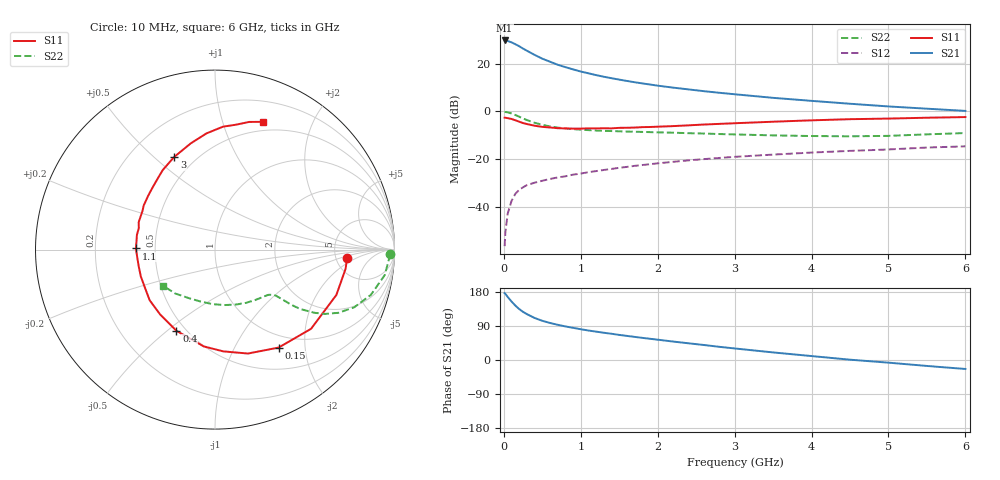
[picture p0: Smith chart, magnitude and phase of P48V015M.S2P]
! SIEMENS Small Signal Semiconductors
! BFP182
! Si NPN RF Bipolar Junction Transistor in SOT143
! VCE = 8 V  IC = 15 mA
! Common Emitter S-Parameters:  March  1996
# GHz  S  MA  R  50
!  f  S11  S21  S12  S22
! GHz  MAG  ANG  MAG  ANG  MAG  ANG  MAG  ANG
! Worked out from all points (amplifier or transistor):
!   36 points, 10 MHz to 6 GHz, reference 50 ohm
!   highest |S21| = 29.7 dB at 10 MHz (marker M1)
!   |S21| within 3 dB of that: start of sweep to 229 MHz
!   unconditionally stable (mu >= 1): 1.087 GHz to 5.576 GHz
!   at 250 MHz: K = 0.39, MSG = 29.1 dB, |S12| = -31.8 dB
!   at 1.4 GHz: K = 1.09, MAG = 17.1 dB, |S12| = -24.1 dB
!   at 6 GHz: K = 0.96, MSG = 7.4 dB, |S12| = -14.7 dB
!   S11 on the Smith chart (normalised r, x): 10 MHz: 6.30, -1.34; 150 MHz: 0.81, -1.53; 400 MHz: 0.45, -0.54; 1.1 GHz: 0.39, +0.01; 3 GHz: 0.38, +0.58; 6 GHz: 0.40, +1.36
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0.01  0.7366 -3.8  30.61 176.5  0.0015 87.4  0.9728 -1.5
0.02  0.7356 -8.3  30.53 174.5  0.0029 86.9  0.9703 -3.3
0.05  0.7218 -20.5  29.87 166.5  0.0072 83.1  0.9565 -8.5
0.1  0.6937 -39.5  27.9 154.3  0.0133 70.7  0.9043 -16.2
0.15  0.6508 -57.0  25.54 143.5  0.0188 64.6  0.8397 -22.5
0.2  0.6075 -72.4  23.12 134.4  0.0227 59.3  0.7729 -27.1
0.25  0.5692 -85.2  20.67 126.9  0.0257 55.2  0.7104 -30.3
0.3  0.5431 -96.6  18.63 121.0  0.0285 53.1  0.6574 -32.4
0.4  0.5008 -115.4  15.26 110.9  0.0321 50.4  0.578 -34.9
0.5  0.4734 -130.2  12.71 103.5  0.0352 48.1  0.523 -35.9
0.6  0.4605 -142.3  10.98 97.7  0.0384 48.3  0.4841 -36.3
0.7  0.4444 -151.4  9.484 92.9  0.0413 48.6  0.4582 -36.6
0.9  0.4353 -167.4  7.577 84.9  0.0473 48.3  0.4245 -37.1
1.1  0.4407 179.2  6.274 77.8  0.0533 48.7  0.4046 -38.5
1.3  0.4427 169.4  5.313 71.9  0.0592 49.0  0.3911 -40.1
1.6  0.4535 156.2  4.344 63.6  0.0687 48.3  0.3777 -43.5
2.2  0.4913 134.9  3.145 48.7  0.0877 45.3  0.358 -52.5
3  0.5642 113.7  2.284 30.5  0.1116 39.3  0.3293 -68.1
3.5  0.6074 102.8  1.922 20.0  0.1243 34.8  0.314 -79.7
4.5  0.6862 86.3  1.445 0.8  0.1487 26.6  0.3003 -105.9
5.5  0.7364 75.0  1.138 -15.7  0.1747 19.3  0.3301 -132.2
6  0.7599 69.5  1.024 -23.7  0.1851 14.6  0.352 -144.8
